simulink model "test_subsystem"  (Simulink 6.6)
settings: Solver=ode45  StartTime=0.0  StopTime=10.0  RelTol=1e-3
libraries: sltpda x6

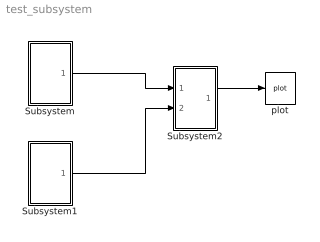
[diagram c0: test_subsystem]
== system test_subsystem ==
  Subsystem : Subsystem
  Subsystem1 : Subsystem
  Subsystem2 : Subsystem
  plot : sltpda/Sinks/plot  Tag=plot  Description=Plot an analysis object.  SystemSampleTime=-1  xscale=linear  yscale=linear
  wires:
  Subsystem/1(Out1) -> Subsystem2/1(In1)
  Subsystem1/1(Out1) -> Subsystem2/2(In2)
  Subsystem2/1(Out1) -> plot/1

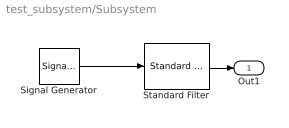
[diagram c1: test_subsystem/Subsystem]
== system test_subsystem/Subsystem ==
  Signal Generator : sltpda/Sources/Signal Generator  Tag=ao  SystemSampleTime=-1  nsecs=10  fs=100  tsfcn=sin(2*pi*10*t)
  Standard Filter : sltpda/Signal Processing blocks/Digital filtering/Standard Filter  Tag=filter  Description=Apply a standard filter type to input AO.  SystemSampleTime=-1  method=filter  ftype=highpass  fgain=1  ffc=0.5  forder=1
  Out1 : Outport
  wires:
  Signal Generator/1 -> Standard Filter/1
  Standard Filter/1 -> Out1/1

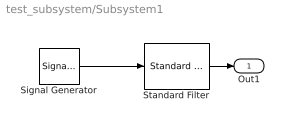
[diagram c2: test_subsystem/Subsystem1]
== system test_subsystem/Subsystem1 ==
  Signal Generator : sltpda/Sources/Signal Generator  Tag=ao  SystemSampleTime=-1  nsecs=10  fs=100  tsfcn=sin(2*pi*1*t)
  Standard Filter : sltpda/Signal Processing blocks/Digital filtering/Standard Filter  Tag=filter  Description=Apply a standard filter type to input AO.  SystemSampleTime=-1  method=filter  ftype=highpass  fgain=1  ffc=0.5  forder=1
  Out1 : Outport
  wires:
  Standard Filter/1 -> Out1/1
  Signal Generator/1 -> Standard Filter/1

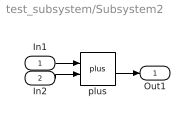
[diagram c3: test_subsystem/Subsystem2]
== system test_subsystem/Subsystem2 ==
  In1 : Inport
  In2 : Inport  Port=2
  plus : sltpda/math blocks/plus  Tag=plus  SystemSampleTime=-1
  Out1 : Outport
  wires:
  In1/1 -> plus/1
  plus/1 -> Out1/1
  In2/1 -> plus/2
